FUNCTION "Gest Posizioni" : VOID
TITLE =Gestione Posizioni
AUTHOR : MassimoZ
FAMILY : NovaSrl
VERSION : 0.1

BEGIN
NETWORK
TITLE =Cont Asse X Crimpatura in Extracorsa +
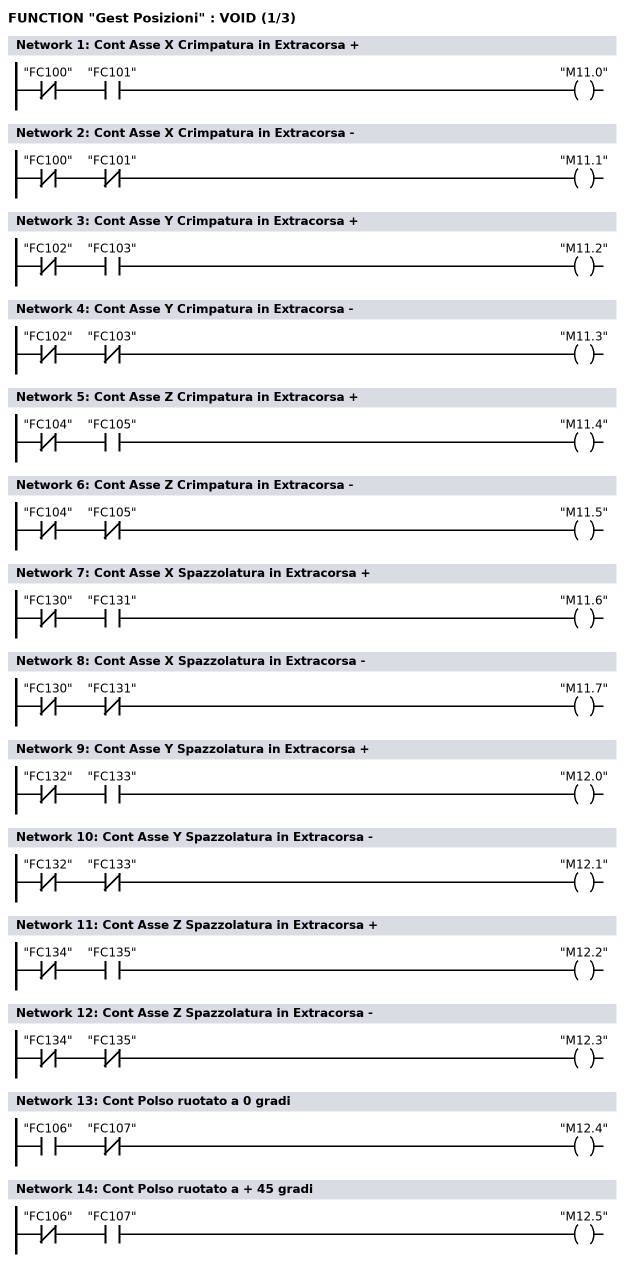
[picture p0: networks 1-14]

      UN    "FC100";
      U     "FC101";
      =     "M11.0";
NETWORK
TITLE =Cont Asse X Crimpatura in Extracorsa -

      UN    "FC100";
      UN    "FC101";
      =     "M11.1";
NETWORK
TITLE =Cont Asse Y Crimpatura in Extracorsa +

      UN    "FC102";
      U     "FC103";
      =     "M11.2";
NETWORK
TITLE =Cont Asse Y Crimpatura in Extracorsa -

      UN    "FC102";
      UN    "FC103";
      =     "M11.3";
NETWORK
TITLE =Cont Asse Z Crimpatura in Extracorsa +

      UN    "FC104";
      U     "FC105";
      =     "M11.4";
NETWORK
TITLE =Cont Asse Z Crimpatura in Extracorsa -

      UN    "FC104";
      UN    "FC105";
      =     "M11.5";
NETWORK
TITLE =Cont Asse X Spazzolatura in Extracorsa +

      UN    "FC130";
      U     "FC131";
      =     "M11.6";
NETWORK
TITLE =Cont Asse X Spazzolatura in Extracorsa -

      UN    "FC130";
      UN    "FC131";
      =     "M11.7";
NETWORK
TITLE =Cont Asse Y Spazzolatura in Extracorsa +

      UN    "FC132";
      U     "FC133";
      =     "M12.0";
NETWORK
TITLE =Cont Asse Y Spazzolatura in Extracorsa -

      UN    "FC132";
      UN    "FC133";
      =     "M12.1";
NETWORK
TITLE =Cont Asse Z Spazzolatura in Extracorsa +

      UN    "FC134";
      U     "FC135";
      =     "M12.2";
NETWORK
TITLE =Cont Asse Z Spazzolatura in Extracorsa -

      UN    "FC134";
      UN    "FC135";
      =     "M12.3";
NETWORK
TITLE =Cont Polso ruotato a 0 gradi

      U     "FC106";
      UN    "FC107";
      =     "M12.4";
NETWORK
TITLE =Cont Polso ruotato a + 45 gradi

      UN    "FC106";
      U     "FC107";
      =     "M12.5";
NETWORK
TITLE =Cont Pinza Crimpatura aperta
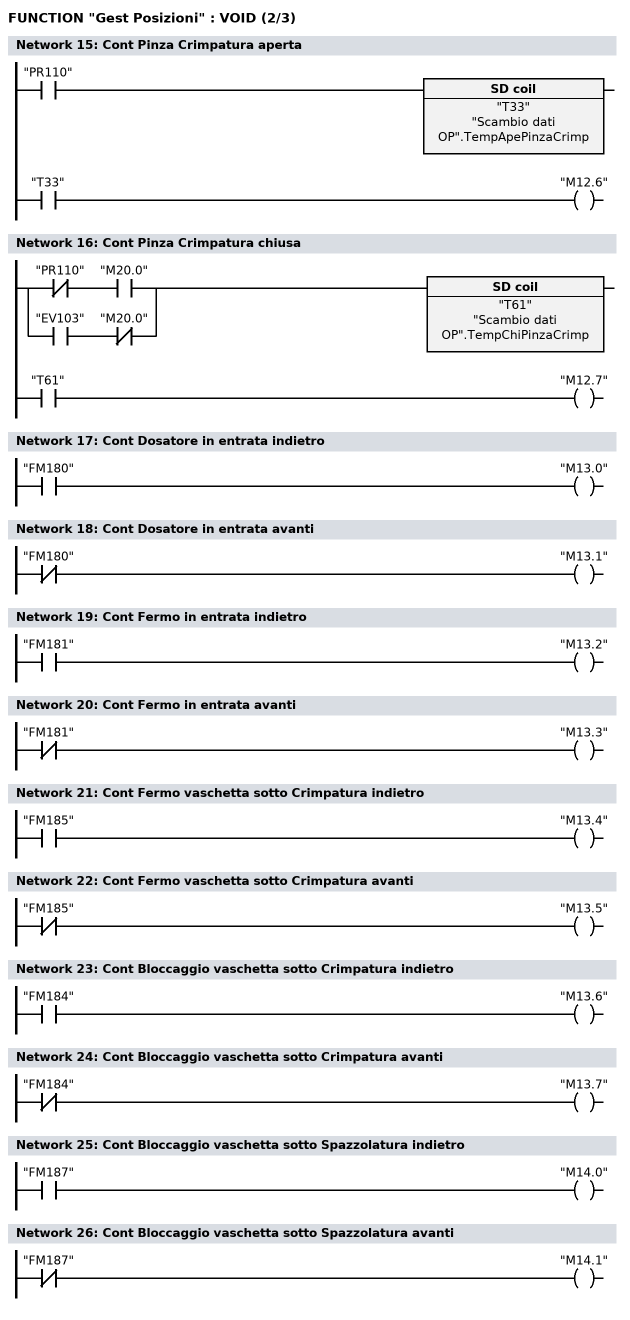
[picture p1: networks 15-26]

      U     "PR110";
      L     "Scambio dati OP".TempApePinzaCrimp;
      SE    "T33";
      NOP   0;
      NOP   0;
      NOP   0;
      U     "T33";
      =     "M12.6";
NETWORK
TITLE =Cont Pinza Crimpatura chiusa

      U(    ;
      UN    "PR110";
      U     "M20.0";
      O     ;
      U     "EV103";
      UN    "M20.0";
      )     ;
      L     "Scambio dati OP".TempChiPinzaCrimp;
      SE    "T61";
      NOP   0;
      NOP   0;
      NOP   0;
      U     "T61";
      =     "M12.7";
NETWORK
TITLE =Cont Dosatore in entrata indietro

      U     "FM180";
      =     "M13.0";
NETWORK
TITLE =Cont Dosatore in entrata avanti

      UN    "FM180";
      =     "M13.1";
NETWORK
TITLE =Cont Fermo in entrata indietro

      U     "FM181";
      =     "M13.2";
NETWORK
TITLE =Cont Fermo in entrata avanti

      UN    "FM181";
      =     "M13.3";
NETWORK
TITLE =Cont Fermo vaschetta sotto Crimpatura indietro

      U     "FM185";
      =     "M13.4";
NETWORK
TITLE =Cont Fermo vaschetta sotto Crimpatura avanti

      UN    "FM185";
      =     "M13.5";
NETWORK
TITLE =Cont Bloccaggio vaschetta sotto Crimpatura indietro

      U     "FM184";
      =     "M13.6";
NETWORK
TITLE =Cont Bloccaggio vaschetta sotto Crimpatura avanti

      UN    "FM184";
      =     "M13.7";
NETWORK
TITLE =Cont Bloccaggio vaschetta sotto Spazzolatura indietro

      U     "FM187";
      =     "M14.0";
NETWORK
TITLE =Cont Bloccaggio vaschetta sotto Spazzolatura avanti

      UN    "FM187";
      =     "M14.1";
NETWORK
TITLE =Cont Fermo vaschetta sotto Spazzolatura indietro
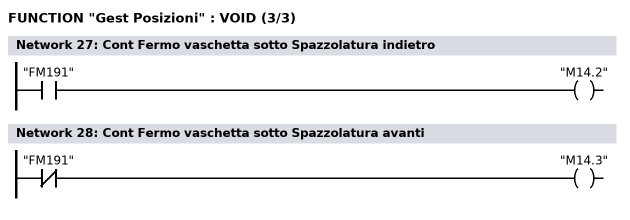
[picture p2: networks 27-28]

      U     "FM191";
      =     "M14.2";
NETWORK
TITLE =Cont Fermo vaschetta sotto Spazzolatura avanti

      UN    "FM191";
      =     "M14.3";
END_FUNCTION

